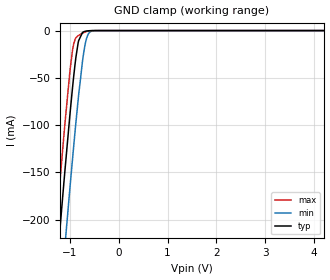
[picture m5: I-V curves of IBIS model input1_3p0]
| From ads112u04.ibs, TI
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|   input1_3p0 Model
[Model]   input1_3p0
Model_type   Input
Vinl = 0.9
Vinh = 2.1
|   typ   min   max
C_comp   6.57107E-13   6.13255E-13   6.94469E-13
[Model spec]
|subparameter
Vinl   0.9   0.8997   0.9003
Vinh   2.1   2.0993   2.1007
| Where Nom  PVT is Nominal Process, 3.0V, 27C
|   Fast PVT is Strong Process,  3.001V, -40C
|   Slow PVT is Weak Process,   2.999, 125C
[Voltage Range]   3   2.999   3.001
[Temperature Range]   27   125   -40
[Power Clamp Reference]   3   2.999   3.001
[GND Clamp Reference]   0   0   0
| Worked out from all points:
|   GND clamp passes 1 mA (typ) near -0.70 V on its own axis
[GND Clamp]
|   Voltage   I(typ)   I(min)   I(max)
-3V       -1.375A    -1.45A     -1.328A
-1.317V   -280.2mA   -360.4mA   -229.6mA
-1.155V   -179.9mA   -259.9mA   -129.7mA
-1.101V   -147.5mA   -227mA     -97.84mA
-1.002V   -90.18mA   -167.9mA   -44.16mA
-930mV    -52.09mA   -126.4mA   -15.99mA
-876mV    -27.77mA   -96.59mA   -7.609mA
-831mV    -12.88mA   -73.02mA   -5.371mA
-723mV    -1.396mA   -25.38mA   -2.299mA
-633mV    -290.5uA   -4.673mA   -671.7uA
-498mV    -12.62uA   -127.9uA   -23.31uA
6V        0A         0A         0A
[POWER Clamp]
|   Voltage   I(typ)   I(min)   I(max)
-3V       0A         0A         0A
0V        0A         0A         0A
6V        0A         0A         0A
